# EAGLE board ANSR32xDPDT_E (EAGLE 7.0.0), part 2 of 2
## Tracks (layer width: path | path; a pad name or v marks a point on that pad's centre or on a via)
GND  (via drill 0.5, 0.9)
  Top 0.254: 289.56,74.82 289.56,76.85 288.93,77.48 | FOR_NANO.GND@1 289.56,69.86 | 284.48,93.99 284.48,87.01
  Top 0.406: C1.2 C4.2 | C3.2 C2.2
  Top 1.016: 289.56,67.45 289.56,73.67 289.56,74.82
  Bottom 0.254: 284.48,88.91 FOR_NANO.GND
  other vias: 226.06,82.56 105.41,82.56 274.95,83.2 311.79,83.83 285.12,84.09 315.6,83.83 299.08,80.02 300.48,76.47 281.56,62.62
  pour Top (isolate 0.305): 322.26,43.83 309.56,43.83 309.56,57.16 322.26,57.16
  pour Top (isolate 0.305): -3.17,95.26 321.31,95.26 321.31,57.16 -3.17,57.16
  pour Bottom (isolate 0.305): -5.08,57.16 -5.08,95.26 321.31,95.26 321.31,57.16
  pour Top (isolate 0.305): 323.53,22.87 309.56,22.87 309.56,55.89 323.53,55.89
  pour Top: 320.99,22.87 310.2,22.87 310.2,55.89 320.99,55.89
I2C_SCL  (via drill 0.5, 0.6, 0.9)
  Top 0.254: v274.95,88.28 268.61,88.28 267.97,87.64 v267.97,78.75 | X26.4 294.26,77.48 294.26,78.12 293.24,79.13 291.08,79.13 290.85,79.37 RN26.3 290.83,83.01 290.83,81.29 v290.19,81.29
  Top 0.305: IC2.12 102.87,78.38 103.77,77.48 106.68,77.48 v107.95,78.75 | v223.52,79.39 IC1.12
  Top 0.406: v274.95,88.28 278.13,88.28 278.76,87.64 278.76,84.47 280.67,82.56 v281.94,82.56
  Bottom 0.254: FOR_NANO.A5 297.18,83.83 303.53,77.48 X26.4
  Bottom 0.305: v267.97,78.75 224.16,78.75 v223.52,79.39 221.62,79.39 220.34,78.12 194.94,78.12 194.31,78.75 110.49,78.75 109.86,79.39 108.58,79.39 v107.95,78.75
  Bottom 0.406: v281.94,82.56 288.93,82.56 v290.19,81.29
I2C_SDA  (via drill 0.5, 0.6, 0.9)
  Top 0.254: v274.95,90.82 267.97,90.82 266.7,89.55 v266.7,77.48 | RN26.4 291.65,82.63 v292.35,81.93 | v292.98,77.47 v292.99,77.48 | X26.3 303.53,80.02 302.26,78.75 v295.27,78.75
  Top 0.305: IC2.13 101.6,77.87 103.25,76.21 107.31,76.21 v109.22,78.12 | v222.25,78.12 IC1.13
  Top 0.406: v274.95,90.82 278.76,90.82 280.04,89.55 280.04,87.01 v281.94,85.1
  Bottom 0.254: v292.35,81.93 292.35,78.12 v292.99,77.48 294.26,78.75 v295.27,78.75 | FOR_NANO.A4 299.72,85.74 305.44,80.02 X26.3
  Bottom 0.305: v109.22,78.12 193.68,78.12 194.31,77.48 221.62,77.48 v222.25,78.12 266.06,78.12 v266.7,77.48
  Bottom 0.406: v281.94,85.1 289.58,85.1 RN26.4 291.65,82.63 v292.35,81.93
N$1
  Bottom 1.27: X1.5 306.07,128.92 306.07,122.11 K9.P2
N$2
  Bottom 1.27: X1.6 304.17,125.74 304.17,119.04 K9.O2
N$3
  Top 2.54: X1.4 308.61,124.83 K9.S2
N$4
  Top 1.27: K9.P1 300.69,119.7 297.81,122.57 297.81,125.74 300.99,128.92 300.99,135.27
  Top 2.54: X1.2 300.99,135.27
N$5
  Top 1.27: K9.O1 300.58,114.72 295.91,119.39 295.91,135.27
  Top 2.54: X1.3 295.91,135.27
N$6
  Top 1.27: 306.07,135.27 306.07,130.19 306.07,129.55 306.07,127.65 303.12,124.7 K9.S1
  Top 2.54: X1.1 306.07,135.27
N$7
  Bottom 1.27: X2.5 290.83,128.92 290.83,122.11 K10.P2
N$8
  Bottom 1.27: X2.6 288.93,125.74 288.93,119.04 K10.O2
N$9
  Top 2.54: X2.4 293.37,124.83 K10.S2
N$10
  Top 1.27: 290.83,135.27 290.83,130.19 290.83,129.55 290.83,127.65 287.88,124.7 K10.S1
  Top 2.54: X2.1 290.83,135.27
N$11
  Top 1.27: K10.P1 285.44,119.7 282.57,122.57 282.57,125.74 285.75,128.92 285.75,135.27
  Top 2.54: X2.2 285.75,135.27
N$12
  Top 1.27: K10.O1 285.34,114.72 280.67,119.39 280.67,135.27
  Top 2.54: X2.3 280.67,135.27
N$13
  Bottom 1.27: X3.5 275.59,128.92 275.59,122.11 K11.P2
N$14
  Bottom 1.27: X3.6 273.69,125.74 273.69,119.04 K11.O2
N$15
  Bottom 1.27: X4.5 260.35,128.92 260.35,122.11 K12.P2
N$16
  Bottom 1.27: X4.6 258.44,125.74 258.44,119.04 K12.O2
N$17
  Top 2.54: X3.4 278.13,124.83 K11.S2
N$18
  Top 2.54: X4.4 262.89,124.83 K12.S2
N$19
  Top 1.27: K11.O1 270.1,114.72 265.43,119.39 265.43,135.27
  Top 2.54: X3.3 265.43,135.27
N$20
  Top 1.27: K12.O1 254.86,114.72 250.19,119.39 250.19,135.27
  Top 2.54: X4.3 250.19,135.27
N$21
  Top 1.27: K12.P1 254.97,119.7 252.09,122.57 252.09,125.74 255.27,128.92 255.27,135.27
  Top 2.54: X4.2 255.27,135.27
N$22
  Top 1.27: K11.P1 270.2,119.7 267.33,122.57 267.33,125.74 270.51,128.92 270.51,135.27
  Top 2.54: X3.2 270.51,135.27
N$23
  Top 1.27: 275.59,135.27 275.59,127.65 272.64,124.7 K11.S1
  Top 2.54: X3.1 275.59,135.27
N$24
  Top 1.27: 260.35,135.27 260.35,127.65 257.4,124.7 K12.S1
  Top 2.54: X4.1 260.35,135.27
N$25
  Bottom 1.27: X5.6 226.06,125.74 226.06,119.04 K13.O2
N$26
  Bottom 1.27: X5.5 227.97,128.92 227.97,122.11 K13.P2
N$27
  Top 2.54: X5.4 230.5,124.83 K13.S2
N$28
  Top 1.27: K13.P1 222.58,119.7 219.71,122.57 219.71,125.74 222.88,128.92 222.88,135.27
  Top 2.54: X5.2 222.88,135.27
N$29
  Top 1.27: 227.97,135.27 227.97,127.65 225.02,124.7 K13.S1
  Top 2.54: X5.1 227.97,135.27
N$30
  Top 1.27: K13.O1 222.48,114.72 217.81,119.39 217.81,135.27
  Top 2.54: X5.3 217.81,135.27
N$31
  Bottom 1.27: X6.5 212.72,128.92 212.72,122.11 K14.P2
N$32
  Bottom 1.27: X6.6 210.82,125.74 210.82,119.04 K14.O2
N$33
  Top 1.27: K14.P1 207.34,119.7 204.47,122.57 204.47,125.74 207.65,128.92 207.65,135.27
  Top 2.54: X6.2 207.65,135.27
N$34
  Top 1.27: 212.72,135.27 212.72,127.65 209.78,124.7 K14.S1
  Top 2.54: X6.1 212.72,135.27
N$35
  Top 1.27: K15.P1 192.1,119.7 189.23,122.57 189.23,125.74 192.41,128.92 192.41,135.27
  Top 2.54: X7.2 192.41,135.27
N$36
  Top 1.27: K16.P1 176.86,119.7 173.99,122.57 173.99,125.74 177.16,128.92 177.16,135.27
  Top 2.54: X8.2 177.16,135.27
N$37
  Bottom 1.27: X8.5 182.25,128.92 182.25,122.11 K16.P2
N$38
  Bottom 1.27: X8.6 180.34,125.74 180.34,119.04 K16.O2
N$39
  Top 1.27: K14.O1 207.65,114.95 202.56,120.03 202.56,135.27
  Top 2.54: X6.3 202.56,135.27
N$40
  Top 1.27: K16.O1 176.76,114.72 172.09,119.39 172.09,135.27
  Top 2.54: X8.3 172.09,135.27
N$41
  Top 1.27: K15.O1 192,114.72 187.32,119.39 187.32,135.27
  Top 2.54: X7.3 187.32,135.27
N$42
  Bottom 1.27: X7.6 195.58,125.74 195.58,119.04 K15.O2
N$43
  Bottom 1.27: X7.5 197.49,128.92 197.49,122.11 K15.P2
N$44
  Top 2.54: X6.4 215.26,124.83 K14.S2
N$45
  Top 2.54: X7.4 200.03,124.83 K15.S2
N$46
  Top 1.27: 197.49,135.27 197.49,127.65 194.54,124.7 K15.S1
  Top 2.54: X7.1 197.49,135.27
N$47
  Top 1.27: 182.25,135.27 182.25,127.65 179.3,124.7 K16.S1
  Top 2.54: X8.1 182.25,135.27
N$48
  Top 2.54: X8.4 184.78,124.83 K16.S2
N$49
  Bottom 1.27: X9.5 139.7,23.51 139.7,30.31 K17.P2
N$50
  Bottom 1.27: X9.6 141.6,26.05 141.6,33.39 K17.O2
N$51
  Top 2.54: X9.4 137.16,27.6 K17.S2
N$52
  Top 1.27: 144.78,17.16 144.78,23.51 147.96,26.68 147.96,29.55 K17.P1
  Top 2.54: X9.2 144.78,17.16
N$53
  Top 1.27: 149.86,17.16 149.86,32.63 K17.O1
  Top 2.54: X9.3 149.86,17.16
N$54
  Top 1.27: K17.S1 144.78,27.32 142.88,27.32 139.7,24.14 139.7,17.16
  Top 2.54: X9.1 139.7,17.16
N$55
  Bottom 1.27: X10.5 127,21.6 124.46,24.14 124.46,30.31 K18.P2
N$56
  Bottom 1.27: X10.6 126.36,26.68 126.36,33.39 K18.O2
N$57
  Top 2.54: X10.4 121.92,27.6 K18.S2
N$58
  Top 1.27: 124.46,17.16 124.46,24.78 127.41,27.72 K18.S1
  Top 2.54: X10.1 124.46,17.16
N$59
  Top 1.27: 129.54,17.16 129.54,23.51 132.72,26.68 132.72,29.55 K18.P1
  Top 2.54: X10.2 129.54,17.16
N$60
  Top 1.27: 134.62,17.16 134.62,32.63 K18.O1
  Top 2.54: X10.3 134.62,17.16
N$61
  Bottom 1.27: X11.5 109.22,23.51 109.22,30.31 K19.P2
N$62
  Bottom 1.27: X11.6 111.12,26.68 111.12,33.39 K19.O2
N$63
  Bottom 1.27: X12.5 93.98,23.51 93.98,30.31 K20.P2
N$64
  Bottom 1.27: X12.6 95.89,26.68 95.89,33.39 K20.O2
N$65
  Top 2.54: X11.4 106.68,27.6 K19.S2
N$66
  Top 2.54: X12.4 91.44,27.6 K20.S2
N$67
  Top 1.27: 119.38,17.16 119.38,32.63 K19.O1
  Top 2.54: X11.3 119.38,17.16
N$68
  Top 1.27: 104.14,17.16 104.14,32.63 K20.O1
  Top 2.54: X12.3 104.14,17.16
N$69
  Top 1.27: 99.06,17.16 99.06,23.51 102.23,26.68 102.23,29.55 K20.P1
  Top 2.54: X12.2 99.06,17.16
N$70
  Top 1.27: 114.3,17.16 114.3,23.51 117.47,26.68 117.47,29.55 K19.P1
  Top 2.54: X11.2 114.3,17.16
N$71
  Top 1.27: 109.22,17.16 109.22,24.78 112.17,27.72 K19.S1
  Top 2.54: X11.1 109.22,17.16
N$72
  Top 1.27: K20.S1 99.06,27.32 97.16,27.32 93.98,24.14 93.98,17.16
  Top 2.54: X12.1 93.98,17.16
N$73
  Bottom 1.27: X13.6 63.5,26.68 63.5,33.39 K21.O2
N$74
  Bottom 1.27: X13.5 61.59,23.51 61.59,30.31 K21.P2
N$75
  Top 2.54: X13.4 59.05,27.6 K21.S2
N$76
  Top 1.27: K21.P1 66.98,32.73 69.85,29.86 69.85,26.68 66.67,23.51 66.67,17.16
  Top 2.54: X13.2 66.67,17.16
N$77
  Top 1.27: K21.S1 66.67,27.32 64.77,27.32 61.59,24.14 61.59,17.16
  Top 2.54: X13.1 61.59,17.16
N$78
  Top 1.27: 71.75,17.16 71.75,32.63 K21.O1
  Top 2.54: X13.3 71.75,17.16
N$79
  Bottom 1.27: X14.5 46.35,23.51 46.35,30.31 K22.P2
N$80
  Bottom 1.27: X14.6 48.26,26.68 48.26,33.39 K22.O2
N$81
  Top 1.27: K22.P1 51.74,32.73 54.61,29.86 54.61,26.68 51.44,23.51 51.44,17.16
  Top 2.54: X14.2 51.44,17.16
N$82
  Top 1.27: K22.S1 51.44,27.32 49.53,27.32 46.35,24.14 46.35,17.16
  Top 2.54: X14.1 46.35,17.16
N$83
  Top 1.27: 36.2,17.16 36.2,23.51 39.37,26.68 39.37,29.55 K23.P1
  Top 2.54: X15.2 36.2,17.16
N$84
  Top 1.27: 20.95,17.16 20.95,23.51 24.13,26.68 24.13,29.55 K24.P1
  Top 2.54: X16.2 20.95,17.16
N$85
  Bottom 1.27: X16.5 15.88,23.51 15.88,30.31 K24.P2
N$86
  Bottom 1.27: X16.6 17.78,26.68 17.78,33.39 K24.O2
N$87
  Top 1.27: K22.O1 51.84,37.71 56.52,33.03 56.52,17.16
  Top 2.54: X14.3 56.52,17.16
N$88
  Top 1.27: 26.04,17.16 26.04,32.63 K24.O1
  Top 2.54: X16.3 26.04,17.16
N$89
  Top 1.27: 41.27,17.16 41.27,32.63 K23.O1
  Top 2.54: X15.3 41.27,17.16
N$90
  Bottom 1.27: X15.6 33.02,26.68 33.02,33.39 K23.O2
N$91
  Bottom 1.27: X15.5 31.11,23.51 31.11,30.31 K23.P2
N$92
  Top 2.54: X14.4 43.81,27.6 K22.S2
N$93
  Top 2.54: X15.4 28.57,27.6 K23.S2
N$94
  Top 1.27: 31.11,17.16 31.11,20.97 31.11,22.64 31.11,24.14 34.7,27.72 K23.S1
  Top 2.54: X15.1 31.11,17.16
N$95
  Top 1.27: 15.88,17.16 15.88,24.14 19.05,27.32 20.32,27.32 20.73,27.72 K24.S1
  Top 2.54: X16.1 15.88,17.16
N$96
  Top 2.54: X16.4 13.34,27.6 K24.S2
N$97
  Bottom 1.27: X17.5 149.86,128.92 149.86,122.11 K25.P2
N$98
  Bottom 1.27: X17.6 147.96,125.74 147.96,119.04 K25.O2
N$99
  Top 2.54: X17.4 152.4,124.83 K25.S2
N$100
  Top 1.27: K25.P1 144.47,119.7 141.6,122.57 141.6,125.74 144.78,128.92 144.78,135.27
  Top 2.54: X17.2 144.78,135.27
N$101
  Top 1.27: K25.O1 144.78,114.95 139.7,120.03 139.7,135.27
  Top 2.54: X17.3 139.7,135.27
N$102
  Top 1.27: 149.86,135.27 149.86,128.28 146.28,124.7 K25.S1
  Top 2.54: X17.1 149.86,135.27
N$103
  Bottom 1.27: X18.5 134.62,128.92 134.62,122.11 K26.P2
N$104
  Bottom 1.27: X18.6 132.72,125.74 132.72,119.04 K26.O2
N$105
  Top 2.54: X18.4 137.16,124.83 K26.S2
N$106
  Top 1.27: 134.62,135.27 134.62,128.28 131.04,124.7 K26.S1
  Top 2.54: X18.1 134.62,135.27
N$107
  Top 1.27: K26.P1 129.24,119.7 126.36,122.57 126.36,125.74 129.54,128.92 129.54,135.27
  Top 2.54: X18.2 129.54,135.27
N$108
  Top 1.27: K26.O1 129.54,114.95 124.46,120.03 124.46,135.27
  Top 2.54: X18.3 124.46,135.27
N$109
  Bottom 1.27: X19.5 119.38,128.92 119.38,122.11 K27.P2
N$110
  Bottom 1.27: X19.6 117.47,125.74 117.47,119.04 K27.O2
N$111
  Bottom 1.27: X20.5 104.14,128.92 104.14,122.11 K28.P2
N$112
  Bottom 1.27: X20.6 102.23,125.74 102.23,119.04 K28.O2
N$113
  Top 2.54: X19.4 121.92,124.83 K27.S2
N$114
  Top 2.54: X20.4 106.68,124.83 K28.S2
N$115
  Top 1.27: K27.O1 113.89,114.72 109.22,119.39 109.22,135.27
  Top 2.54: X19.3 109.22,135.27
N$116
  Top 1.27: K28.O1 98.65,114.72 93.98,119.39 93.98,135.27
  Top 2.54: X20.3 93.98,135.27
N$117
  Top 1.27: K28.P1 98.75,119.7 95.89,122.57 95.89,125.74 99.06,128.92 99.06,135.27
  Top 2.54: X20.2 99.06,135.27
N$118
  Top 1.27: K27.P1 113.36,119.7 111.12,121.93 111.12,125.74 114.3,128.92 114.3,135.27
  Top 2.54: X19.2 114.3,135.27
N$119
  Top 1.27: 119.38,135.27 119.38,128.28 115.8,124.7 K27.S1
  Top 2.54: X19.1 119.38,135.27
N$120
  Top 1.27: 104.14,135.27 104.14,128.28 100.56,124.7 K28.S1
  Top 2.54: X20.1 104.14,135.27
N$121
  Bottom 1.27: K29.O2 73.89,114.72 69.85,118.76 69.85,125.74 X21.6
N$122
  Bottom 1.27: K29.P2 73.99,119.7 71.75,121.93 71.75,128.92 X21.5
N$123
  Top 2.54: X21.4 74.3,124.83 K29.S2
N$124
  Top 1.27: K29.P1 66.37,119.7 63.5,122.57 63.5,125.74 66.67,128.92 66.67,135.27
  Top 2.54: X21.2 66.67,135.27
N$125
  Top 1.27: 71.75,135.27 71.75,128.28 68.17,124.7 K29.S1
  Top 2.54: X21.1 71.75,135.27
N$126
  Top 1.27: K29.O1 66.27,114.72 61.59,119.39 61.59,135.27
  Top 2.54: X21.3 61.59,135.27
N$127
  Bottom 1.27: K30.P2 58.93,120.15 56.52,122.57 56.52,128.92 X22.5
N$128
  Bottom 1.27: K30.O2 58.65,114.72 54.61,118.76 54.61,125.74 X22.6
N$129
  Top 1.27: K30.P1 51.13,119.7 48.26,122.57 48.26,125.74 51.44,128.92 51.44,135.27
  Top 2.54: X22.2 51.44,135.27
N$130
  Top 1.27: 56.52,135.27 56.52,128.28 52.93,124.7 K30.S1
  Top 2.54: X22.1 56.52,135.27
N$131
  Top 1.27: K31.P1 36.2,120.03 33.02,123.2 33.02,125.74 36.2,128.92 36.2,135.27
  Top 2.54: X23.2 36.2,135.27
N$132
  Top 1.27: K32.P1 20.95,120.03 17.78,123.2 17.78,125.74 20.95,128.92 20.95,135.27
  Top 2.54: X24.2 20.95,135.27
N$133
  Bottom 1.27: K32.P2 28.45,120.15 26.04,122.57 26.04,128.92 X24.5
N$134
  Bottom 1.27: K32.O2 28.17,114.72 24.13,118.76 24.13,125.74 X24.6
N$135
  Top 1.27: K30.O1 51.03,114.72 46.35,119.39 46.35,135.27
  Top 2.54: X22.3 46.35,135.27
N$136
  Top 1.27: K32.O1 20.55,114.72 15.88,119.39 15.88,135.27
  Top 2.54: X24.3 15.88,135.27
N$137
  Top 1.27: K31.O1 36.2,114.95 31.11,120.03 31.11,135.27
  Top 2.54: X23.3 31.11,135.27
N$138
  Bottom 1.27: K31.O2 43.69,115.07 39.37,119.39 39.37,125.74 X23.6
N$139
  Bottom 1.27: K31.P2 43.69,120.15 41.27,122.57 41.27,128.92 X23.5
N$140
  Top 2.54: X22.4 59.05,124.83 K30.S2
N$141
  Top 2.54: X23.4 43.81,124.83 K31.S2
N$142
  Top 1.27: 41.27,135.27 41.27,128.28 37.69,124.7 K31.S1
  Top 2.54: X23.1 41.27,135.27
N$143
  Top 1.27: 26.04,135.27 26.04,128.28 22.45,124.7 K32.S1
  Top 2.54: X24.1 26.04,135.27
N$144
  Top 2.54: X24.4 28.57,124.83 K32.S2
N$163
  Top 0.254: POWER1.A 317.11,30.61 316.74,30.24 315.46,30.24 RNB1.3
  Top 0.406: 315.42,30.37 RNB1.3
N$164
  Top 0.813: 282.57,66.18 IC7.8 291.01,66.18 H1.2 | 282.57,66.18 280.8,66.18 280.04,65.42 280.04,60.87 279.53,60.36 279.53,58.96 D1.C 279.38,58.81 277.37,58.81 276.48,59.7 269.24,59.7 268.35,60.59 CD1.2 | 282.55,66.2 282.57,66.18
N$165
  Top 0.813: CD1.1 270.66,67.17 271.78,66.05 276.61,66.05 276.73,66.18 IC7.1
N$203
  Bottom 1.27: X28.5 295.91,23.51 295.91,30.31 K1.P2
N$204
  Bottom 1.27: X28.6 297.81,26.05 297.81,32.75 K1.O2
N$205
  Top 2.54: X28.4 293.37,27.6 K1.S2
N$206
  Top 1.27: K1.P1 301.3,32.73 304.17,29.86 304.17,26.68 300.99,23.51 300.99,17.16
  Top 2.54: X28.2 300.99,17.16
N$207
  Top 1.27: K1.O1 300.99,37.48 306.07,32.4 306.07,17.16
  Top 2.54: X28.3 306.07,17.16
N$208
  Top 1.27: 295.91,17.16 295.91,24.78 298.86,27.72 K1.S1
  Top 2.54: X28.1 295.91,17.16
N$209
  Bottom 1.27: X29.5 280.67,23.51 280.67,30.31 K2.P2
N$210
  Bottom 1.27: X29.6 282.57,26.68 282.57,33.39 K2.O2
N$211
  Top 2.54: X29.4 278.13,27.6 K2.S2
N$212
  Top 1.27: K2.S1 285.75,27.32 283.85,27.32 280.67,24.14 280.67,17.16
  Top 2.54: X29.1 280.67,17.16
N$213
  Top 1.27: K2.P1 286.06,32.73 288.93,29.86 288.93,26.68 285.75,23.51 285.75,17.16
  Top 2.54: X29.2 285.75,17.16
N$214
  Top 1.27: K2.O1 285.75,37.48 290.83,32.4 290.83,17.16
  Top 2.54: X29.3 290.83,17.16
N$215
  Bottom 1.27: X30.5 265.43,23.51 265.43,30.31 K3.P2
N$216
  Bottom 1.27: X30.6 267.33,26.68 267.33,33.39 K3.O2
N$217
  Bottom 1.27: X31.5 252.09,20.97 250.19,22.87 250.19,30.31 K4.P2
N$218
  Bottom 1.27: X31.6 252.09,26.68 252.09,33.39 K4.O2
N$219
  Top 2.54: X30.4 262.89,27.6 K3.S2
N$220
  Top 2.54: X31.4 247.78,20.97 K4.S2
N$221
  Top 1.27: K3.O1 270.92,37.71 275.59,33.03 275.59,17.16
  Top 2.54: X30.3 275.59,17.16
N$222
  Top 1.27: 260.35,17.16 260.35,32.63 K4.O1
  Top 2.54: X31.3 260.35,17.16
N$223
  Top 1.27: K4.P1 255.27,32.4 258.44,29.22 258.44,26.68 255.27,23.51 255.27,17.16
  Top 2.54: 255.27,17.16 X31.2
N$224
  Top 1.27: 270.51,17.16 270.51,23.51 273.69,26.68 273.74,29.48 273.38,29.86 K3.P1
  Top 2.54: X30.2 270.51,17.16
N$225
  Top 1.27: 265.43,17.16 265.43,24.78 268.38,27.72 K3.S1
  Top 2.54: X30.1 265.43,17.16
N$226
  Top 1.27: 250.19,17.16 250.19,24.78 253.14,27.72 K4.S1
  Top 2.54: X31.1 250.19,17.16
N$304
  Bottom 1.27: X32.6 219.71,26.68 219.71,33.39 K5.O2
N$305
  Bottom 1.27: X32.5 217.81,23.51 217.81,30.31 K5.P2
N$306
  Top 2.54: X32.4 215.26,27.6 K5.S2
N$307
  Top 1.27: 222.88,17.16 222.88,23.51 226.06,26.68 226.06,29.55 K5.P1
  Top 2.54: X32.2 222.88,17.16
N$308
  Top 1.27: 217.81,17.16 217.81,24.78 220.75,27.72 K5.S1
  Top 2.54: X32.1 217.81,17.16
N$309
  Top 1.27: 227.97,17.16 227.97,32.63 K5.O1
  Top 2.54: X32.3 227.97,17.16
N$310
  Bottom 1.27: X33.5 202.56,23.51 202.56,30.31 K6.P2
N$311
  Bottom 1.27: X33.6 204.47,26.68 204.47,33.39 K6.O2
N$312
  Top 1.27: 207.65,17.16 207.65,23.51 210.82,26.68 210.82,29.55 K6.P1
  Top 2.54: X33.2 207.65,17.16
N$313
  Top 1.27: 202.56,17.16 202.56,24.78 205.51,27.72 K6.S1
  Top 2.54: X33.1 202.56,17.16
N$314
  Top 1.27: 192.41,17.16 192.41,23.51 195.58,26.68 195.58,29.55 K7.P1
  Top 2.54: X34.2 192.41,17.16
N$315
  Top 1.27: 177.16,17.16 177.16,23.51 180.34,26.68 180.34,29.55 K8.P1
  Top 2.54: X35.2 177.16,17.16
N$316
  Bottom 1.27: X35.5 172.09,23.51 172.09,30.31 K8.P2
N$317
  Bottom 1.27: X35.6 173.99,26.68 173.99,33.39 K8.O2
N$318
  Top 1.27: 212.72,17.16 212.72,32.63 K6.O1
  Top 2.54: X33.3 212.72,17.16
N$319
  Top 1.27: 182.25,17.16 182.25,32.63 K8.O1
  Top 2.54: X35.3 182.25,17.16
N$320
  Top 1.27: 197.49,17.16 197.49,32.63 K7.O1
  Top 2.54: X34.3 197.49,17.16
N$321
  Bottom 1.27: X34.6 189.23,26.68 189.23,33.39 K7.O2
N$322
  Bottom 1.27: X34.5 187.32,23.51 187.32,30.31 K7.P2
N$323
  Top 2.54: X33.4 200.03,27.6 K6.S2
N$324
  Top 2.54: X34.4 184.78,27.6 K7.S2
N$325
  Top 1.27: 187.32,17.16 187.32,24.78 190.27,27.72 K7.S1
  Top 2.54: X34.1 187.32,17.16
N$326
  Top 1.27: 172.09,17.16 172.09,24.78 175.03,27.72 K8.S1
  Top 2.54: X35.1 172.09,17.16
N$327
  Top 2.54: X35.4 169.54,27.6 K8.S2
N$405  (via drill 0.5)
  Top 0.229: IC1.21 228.6,70.81 227.97,70.18 214.63,70.18 214,70.81 IC3.1
  Top 0.254: 228.6,70.81 v228.6,73.29 | v242.82,70.37 243.46,69.74 245.52,69.74
  Top 0.305: 245.52,69.74 245.58,69.74 RN19.5
  Bottom 0.229: v228.6,73.29 228.6,73.04 229.24,73.67 242.19,73.67 242.82,73.04 v242.82,70.37
N$406  (via drill 0.5)
  Top 0.229: IC1.25 v233.68,69.99 233.68,68.28 233.04,67.64 209.55,67.64 208.91,68.28 IC3.5 | v239.4,66.37 242.89,66.37 243.21,66.05 245.51,66.05 RN18.5
  Bottom 0.229: v233.68,69.99 233.68,71.28 234.04,71.64 238.99,71.64 239.4,71.24 v239.4,66.37
N$407  (via drill 0.5)
  Top 0.229: IC1.26 v234.95,69.99 234.95,67.96 234,67.01 208.28,67.01 207.65,67.64 IC3.6 | v240.35,65.42 242.89,65.42 243.21,65.1 245.5,65.1 RN18.6
  Bottom 0.229: v234.95,69.99 234.95,71.01 235.08,71.13 238.25,71.13 238.38,71.01 238.38,65.67 238.63,65.42 v240.35,65.42
N$408  (via drill 0.6)
  Top 0.305: IC2.16 v101.6,74.94 | v222.25,73.67 IC1.16 | RN17.6 264.05,82.16 | U$13.A1 264.8,90.18 265.43,89.55 265.43,82.56 265.03,82.16 264.05,82.16 | 264.05,82.16 264.92,81.29 v264.92,74.31
  Bottom 0.305: v101.6,74.94 102.87,76.21 110.49,76.21 111.12,76.85 192.41,76.85 193.04,76.21 219.07,76.21 221.62,73.67 v222.25,73.67 222.88,74.31 v264.92,74.31
N$409  (via drill 0.5)
  Top 0.229: IC1.22 229.87,70.18 229.24,69.54 213.36,69.54 212.72,70.18 IC3.2
  Top 0.254: 229.87,70.18 v229.87,69.99 | v241.81,69.61 242.32,69.61 242.95,68.97 245.56,68.97 RN19.6
  Bottom 0.229: v229.87,69.99 229.87,72.78 230.25,73.16 241.3,73.16 241.81,72.66 v241.81,69.61
N$410  (via drill 0.5)
  Top 0.229: IC1.23 231.14,69.54 230.5,68.91 212.09,68.91 211.46,69.54 IC3.3
  Top 0.254: 231.14,69.54 v231.14,69.99 | v240.92,68.59 241.55,68.59 241.94,68.21 245.56,68.21 RN19.7
  Bottom 0.229: v231.14,69.99 231.14,72.4 231.39,72.66 240.54,72.66 240.92,72.28 v240.92,68.59
  Bottom 0.254: 241.17,68.47 v240.92,68.59
N$411  (via drill 0.5)
  Top 0.229: IC1.24 232.41,68.91 231.78,68.28 210.82,68.28 210.19,68.91 IC3.4
  Top 0.254: 232.41,68.91 v232.41,69.99 | v240.54,67.32 245.51,67.32 RN19.8
  Bottom 0.229: v232.41,69.99 232.41,71.64 232.92,72.15 239.27,72.15 240.03,71.39 240.03,67.83 v240.54,67.32
N$416  (via drill 0.6)
  Top 0.203: 212.72,79.39 213.04,79.7 218.76,79.7 219.71,80.66 219.71,82.88 220.34,83.51 236.85,83.51 237.49,84.15 v237.49,88.91
  Top 0.229: v237.49,88.91 237.49,89.8 236.73,90.56 236.73,91.34 RN21.8
  Top 0.406: v237.49,82.56 IC1.1 | IC4.8 212.72,79.39
  Bottom 0.406: v237.49,88.91 v237.49,82.56
N$417  (via drill 0.6)
  Top 0.203: IC4.7 211.46,79.7 211.96,80.21 218.25,80.21 219.07,81.04 219.07,83.51 219.71,84.15 235.59,84.15 236.22,84.78 v236.22,88.91
  Top 0.229: v236.22,88.91 236.22,89.93 235.84,90.31 235.84,91.4 RN21.7
  Top 0.406: v236.22,82.56 IC1.2
  Bottom 0.406: v236.22,88.91 v236.22,82.56
N$418  (via drill 0.6)
  Top 0.203: IC4.6 210.19,80.02 210.88,80.72 217.49,80.72 218.44,81.67 218.44,84.15 219.07,84.78 234.31,84.78 234.95,85.42 v234.95,88.91
  Top 0.229: v234.95,88.91 234.95,90.44 235.08,90.56 235.08,91.4 RN21.6
  Top 0.406: v234.95,82.56 IC1.3
  Bottom 0.406: v234.95,88.91 v234.95,82.56
N$419  (via drill 0.6)
  Top 0.203: IC4.5 208.91,80.02 210.12,81.23 216.85,81.23 217.81,82.18 217.81,84.78 218.44,85.42 233.04,85.42 233.68,86.06 v233.68,88.91
  Top 0.229: v233.68,88.91 233.68,90.06 234.19,90.56 234.19,91.34 RN21.5
  Top 0.406: v233.68,82.56 IC1.4
  Bottom 0.406: v233.68,82.56 v233.68,88.91
N$420  (via drill 0.6)
  Top 0.203: IC4.4 207.65,80.02 209.36,81.74 216.34,81.74 217.17,82.56 217.17,85.42 217.81,86.06 231.78,86.06 232.41,86.69 v232.41,88.91
  Top 0.229: v232.41,88.91 232.41,89.67 231.78,90.31 231.78,91.34 RN20.8
  Top 0.406: v232.41,82.56 IC1.5
  Bottom 0.406: v232.41,88.91 v232.41,82.56
N$421  (via drill 0.6)
  Top 0.203: IC4.3 206.38,80.02 208.6,82.25 215.84,82.25 216.53,82.94 216.53,86.06 217.17,86.69 230.5,86.69 231.14,87.32 v231.14,88.91
  Top 0.229: v231.14,88.91 231.14,90.06 230.89,90.31 230.89,91.4 RN20.7
  Top 0.406: v231.14,82.56 IC1.6
  Bottom 0.406: v231.14,88.91 v231.14,82.56
N$422  (via drill 0.6)
  Top 0.203: IC4.2 205.1,80.02 207.84,82.75 215.2,82.75 215.9,83.45 215.9,86.69 216.53,87.32 229.42,87.32 229.87,87.77 v229.87,88.91
  Top 0.229: IC1.7 229.87,80.66 | v229.87,88.91 229.87,89.93 230.12,90.18 230.12,91.4 RN20.6
  Top 0.406: 229.87,88.54 v229.87,88.91 | v229.87,82.56 IC1.7
  Bottom 0.406: v229.87,88.91 v229.87,82.56
N$423  (via drill 0.6)
  Top 0.203: IC4.1 203.84,80.02 207.2,83.39 214.69,83.39 215.26,83.96 215.26,87.25 215.97,87.96 228.15,87.96 228.6,88.41 v228.6,88.91
  Top 0.229: v228.6,88.91 228.6,89.93 229.24,90.56 229.24,91.34 RN20.5
  Top 0.406: v228.6,82.56 IC1.8
  Bottom 0.406: v228.6,82.56 v228.6,88.91
N$424  (via drill 0.5)
  Top 0.229: IC2.21 v107.95,73.23 107.95,70.76 107.56,70.37 94.61,70.37 93.98,71.01 IC5.1 | v123.19,67.32 124.86,67.32 RN22.5
  Bottom 0.229: v107.95,73.23 107.95,74.31 108.58,74.94 122.56,74.94 123.19,74.31 v123.19,67.32
N$425  (via drill 0.5)
  Top 0.229: IC5.2 92.71,70.5 93.34,69.86 109.22,69.86 v109.22,70.05 IC2.22 | RN22.6 122,66.45 v121.92,66.37
  Bottom 0.229: v121.92,66.37 121.92,73.67 121.28,74.31 109.86,74.31 109.22,73.67 v109.22,70.05
N$426  (via drill 0.5)
  Top 0.229: IC5.3 91.44,69.86 92.08,69.23 109.98,69.23 110.49,69.74 v110.49,70.05 IC2.23 | RN22.7 122.79,65.65 122.56,65.42 v120.65,65.42
  Bottom 0.229: v120.65,65.42 120.65,73.04 120.02,73.67 111.12,73.67 110.49,73.04 v110.49,70.05
N$427  (via drill 0.5)
  Top 0.229: IC5.4 90.17,69.23 90.81,68.59 111.12,68.59 111.76,69.23 v111.76,70.05 IC2.24 | RN22.8 122.94,64.85 122.56,64.47 119.7,64.47 v119.06,65.1
  Bottom 0.229: v119.06,65.1 119.06,72.33 118.35,73.04 112.39,73.04 111.76,72.4 v111.76,70.05
N$428  (via drill 0.5)
  Top 0.229: IC5.5 88.9,68.59 89.53,67.96 112.39,67.96 113.03,68.59 v113.03,70.05 IC2.25 | RN23.5 122.94,63.44 v122.87,63.51
  Bottom 0.229: v122.87,63.51 119.06,63.51 118.11,64.47 118.11,71.77 117.47,72.4 113.67,72.4 113.03,71.77 v113.03,70.05
N$429  (via drill 0.5)
  Top 0.229: IC5.6 87.63,67.96 88.27,67.32 113.67,67.32 114.3,67.96 v114.3,70.05 IC2.26 | RN23.6 122,62.64 v121.92,62.56
  Bottom 0.229: v121.92,62.56 118.75,62.56 117.16,64.15 117.16,71.06 116.45,71.77 114.64,71.77 IC2.26 v114.3,70.05
N$430  (via drill 0.5)
  Top 0.229: IC5.7 86.36,67.32 87,66.69 114.94,66.69 115.57,67.32 v115.57,70.05 IC2.27 | RN23.7 122.79,61.84 122.56,61.61 v120.65,61.61
  Bottom 0.229: v120.65,61.61 117.47,61.61 115.57,63.51 v115.57,70.05
N$431
  Top 0.229: IC2.28 116.84,66.69 | 116.84,66.69 116.2,66.05 85.72,66.05 85.09,66.69 IC5.8 | RN23.8 121.67,61.04 121.28,60.65 119.7,60.65 119.38,60.97 119.38,63.51 116.84,66.05 116.84,66.69
N$432  (via drill 0.6)
  Top 0.203: IC6.8 92.71,79.39 93.34,80.02 98.42,80.02 99.06,80.66 99.06,82.56 100.33,83.83 116.2,83.83 116.84,84.47 v116.84,88.91 | v116.84,82.56 IC2.1
  Top 0.229: v116.84,88.91 116.84,89.87 116.2,90.5 116.2,91.22 RN25.8
  Bottom 0.203: v116.84,88.91 v116.84,82.56
N$433  (via drill 0.6)
  Top 0.203: IC6.7 91.44,79.39 92.46,80.4 97.54,80.4 98.42,81.29 98.42,83.2 99.69,84.47 114.94,84.47 115.57,85.1 v115.57,88.91 | v115.57,82.56 IC2.2
  Top 0.229: v115.57,88.91 115.57,90.18 115.25,90.5 115.25,91.2 RN25.7
  Bottom 0.203: v115.57,88.91 v115.57,82.56
N$434  (via drill 0.6)
  Top 0.203: IC6.6 90.17,79.39 91.57,80.78 96.65,80.78 97.79,81.93 97.79,83.83 99.06,85.1 113.67,85.1 114.3,85.74 v114.3,88.91 | v114.3,82.56 IC2.3
  Top 0.229: v114.3,88.91 114.3,90.18 114.62,90.5 114.62,91.2 RN25.6
  Bottom 0.203: v114.3,88.91 v114.3,82.56
N$435  (via drill 0.6)
  Top 0.203: IC6.5 88.9,80.02 90.04,81.17 95.76,81.17 97.16,82.56 97.16,84.47 98.42,85.74 112.39,85.74 113.03,86.37 v113.03,88.91 | v113.03,82.56 IC2.4
  Top 0.229: v113.03,88.91 113.03,89.87 113.67,90.5 113.67,91.22 RN25.5
  Bottom 0.203: v113.03,88.91 v113.03,82.56
N$436  (via drill 0.6)
  Top 0.203: IC6.4 87.63,80.02 89.15,81.55 94.87,81.55 96.52,83.2 96.52,85.1 97.79,86.37 111.12,86.37 111.76,87.01 v111.76,88.91 | v111.76,82.56 IC2.5
  Top 0.229: v111.76,88.91 111.76,89.87 111.12,90.5 111.12,91.22 RN24.8
  Bottom 0.203: v111.76,88.91 v111.76,82.56
N$437  (via drill 0.6)
  Top 0.203: IC6.3 86.36,80.02 88.27,81.93 93.98,81.93 95.89,83.83 95.89,85.74 97.16,87.01 109.86,87.01 110.49,87.64 v110.49,88.91 | v110.49,82.56 IC2.6
  Top 0.229: v110.49,88.91 110.49,90.18 110.17,90.5 110.17,91.2 RN24.7
  Bottom 0.203: v110.49,88.91 v110.49,82.56
N$438  (via drill 0.6)
  Top 0.203: IC6.2 85.09,80.02 87.38,82.31 93.09,82.31 95.25,84.47 95.25,86.37 96.52,87.64 108.58,87.64 109.22,88.28 v109.22,88.91 | v109.22,82.56 IC2.7
  Top 0.229: v109.22,88.91 109.22,90.18 109.54,90.5 109.54,91.2 RN24.6
  Bottom 0.203: v109.22,88.91 v109.22,82.56
N$439  (via drill 0.6)
  Top 0.203: IC6.1 83.82,80.02 86.49,82.69 92.46,82.69 94.61,84.85 94.61,87.01 95.89,88.28 107.31,88.28 v107.95,88.91 | v107.95,82.56 IC2.8
  Top 0.229: v107.95,88.91 107.95,89.87 108.58,90.5 108.58,91.22 RN24.5
  Bottom 0.203: v107.95,88.91 v107.95,82.56
N$440
  Top 0.406: RN2.7 53.74,82.16 52.7,83.2 34.17,83.2 R30.C
N$441
  Top 0.406: RN5.1 184.22,83.76 183.51,84.47 157.37,84.47 R16.C
N$442
  Top 0.406: RN8.7 RN7.2
N$443
  Top 0.406: RN7.3 RN8.6
N$444
  Top 0.406: RN8.5 RN7.4
N$445
  Top 0.406: RN5.2 183.75,82.96 182.88,83.83 160.54,83.83 R15.C
N$446
  Top 0.406: RN4.3 52.47,78.35 50.16,80.66 46.88,80.66 R26.C
N$447
  Top 0.406: RN5.4 182.81,81.36 181.61,82.56 166.89,82.56 R13.C
N$448
  Top 0.406: RN5.5 RN6.4
N$449
  Top 0.406: RN7.1 RN8.8
N$450
  Top 0.406: RN8.1 182.95,79.95 180.97,81.93 170.06,81.93 R12.C
N$451
  Top 0.406: RN5.6 RN6.3
N$452
  Top 0.406: RN8.2 182.48,79.15 180.34,81.29 173.24,81.29 R11.C
N$453
  Top 0.406: RN6.2 RN5.7
N$454
  Top 0.406: RN5.8 RN6.1
N$455
  Top 0.406: RN3.4 RN4.5
N$456
  Top 0.406: RN2.5 54.68,83.76 53.98,84.47 27.82,84.47 R32.C
N$458
  Top 0.406: RN5.3 183.28,82.16 182.25,83.2 163.72,83.2 R14.C
N$459
  Top 0.406: RN8.3 182.01,78.35 179.71,80.66 176.41,80.66 R10.C
N$460
  Top 0.406: RN2.8 53.27,81.36 52.07,82.56 37.35,82.56 R29.C
N$461
  Top 0.406: RN4.1 53.41,79.95 51.44,81.93 40.52,81.93 R28.C
N$462
  Top 0.406: RN4.2 52.94,79.15 50.8,81.29 43.7,81.29 R27.C
N$463
  Top 0.406: RN12.4 RN11.5
N$464
  Top 0.305: R25.C 49.65,79.39
  Top 0.406: RN4.4 52,77.55 50.16,79.39 49.65,79.39
N$465
  Top 0.406: RN2.1 RN1.8
N$466
  Top 0.406: RN2.2 RN1.7
N$467
  Top 0.406: RN2.3 RN1.6
N$468
  Top 0.406: RN2.4 RN1.5
N$469
  Top 0.406: RN2.6 54.21,82.96 53.34,83.83 31,83.83 R31.C
N$470
  Top 0.406: RN8.4 181.54,77.55 179.71,79.39 179.19,79.39 R9.C
N$473
  Top 0.406: RN12.5 181.54,74.87 179.71,73.04 179.19,73.04 R1.C
N$474
  Top 0.406: RN11.6 RN12.3
N$475
  Top 0.406: RN12.6 182.01,74.07 179.71,71.77 176.41,71.77 R2.C
N$476
  Top 0.406: RN12.7 182.48,73.27 180.34,71.13 173.24,71.13 R3.C
N$477
  Top 0.406: RN9.4 RN10.5
N$478
  Top 0.406: RN10.6 RN9.3
N$479
  Top 0.406: RN9.2 RN10.7
N$480
  Top 0.406: RN10.8 RN9.1
N$481
  Top 0.406: RN12.2 RN11.7
N$482
  Top 0.406: RN10.1 182.81,71.06 181.61,69.86 166.89,69.86 R5.C
N$483
  Top 0.406: RN12.8 182.95,72.47 180.97,70.5 170.06,70.5 R4.C
N$484
  Top 0.406: RN10.3 183.75,69.46 182.88,68.59 160.54,68.59 R7.C
N$485
  Top 0.406: RN10.4 184.22,68.66 183.51,67.96 157.37,67.96 R8.C
N$486
  Top 0.406: RN10.2 183.28,70.26 182.25,69.23 163.72,69.23 R6.C
N$487
  Top 0.406: RN14.3 53.58,73.27 51.44,71.13 43.7,71.13 R19.C
N$488
  Top 0.406: RN14.2 53.1,74.07 50.8,71.77 46.88,71.77 R18.C
N$489
  Top 0.406: RN14.1 52.63,74.87 50.8,73.04 49.65,73.04 R17.C
N$490
  Top 0.406: RN16.4 55.31,68.66 54.61,67.96 27.82,67.96 R24.C
N$491
  Top 0.406: RN15.3 RN16.6
N$492
  Top 0.406: RN15.2 RN16.7
N$493
  Top 0.406: RN15.1 62.8,71.06 62.87,71.13 58.02,71.13 RN16.8
N$494
  Top 0.406: RN14.4 54.05,72.47 52.07,70.5 40.52,70.5 R20.C
N$495
  Top 0.406: RN16.3 54.84,69.46 53.98,68.59 31,68.59 R23.C
N$496
  Top 0.406: RN16.2 54.38,70.26 53.34,69.23 34.17,69.23 R22.C
N$497
  Top 0.406: RN16.1 53.91,71.06 52.7,69.86 37.35,69.86 R21.C
N$498  (via drill 0.6)
  Top 0.305: IC2.17 v102.87,73.67 | v219.07,73.67 219.07,74.94 219.71,75.58 v222.25,75.58 222.88,75.58 223.52,74.94 IC1.17 | U$13.B1 261.62,86.37 261.62,81.29 261.69,81.36 RN17.5 263.14,81.36 263.84,80.66 v263.84,75.58
  Bottom 0.305: v102.87,73.67 104.78,75.58 111.12,75.58 111.76,76.21 191.83,76.21 192.41,75.58 218.44,75.58 219.07,74.94 v219.07,73.67 | v222.25,75.58 v263.84,75.58
N$500
  Top 0.406: RN11.8 RN12.1
N$501
  Top 0.406: RN13.4 RN14.5
N$502
  Top 0.406: RN14.6 RN13.3
N$503
  Top 0.406: RN13.2 RN14.7
N$504
  Top 0.406: RN14.8 RN13.1
N$505
  Top 0.406: RN4.6 RN3.3
N$506
  Top 0.406: RN4.7 RN3.2
N$507
  Top 0.406: RN4.8 RN3.1
N$514
  Top 0.406: RN15.4 RN16.5
N$525  (via drill 0.5)
  Top 0.229: IC3.7 206.38,67.01 207.01,66.37 235.27,66.37 236.22,67.32 v236.22,69.99 IC1.27 | v241.3,64.47 245.03,64.47 RN18.7
  Bottom 0.229: v241.3,64.47 236.54,64.47 236.22,64.78 v236.22,69.99
N$526
  Top 0.229: IC1.28 237.49,66.37 | 237.49,66.37 236.85,65.73 205.74,65.73 205.1,66.37 IC3.8 | 237.49,66.37 237.49,64.15 238.12,63.51 245.51,63.51 RN18.8
OC_R1_A  (via drill 0.6)
  Top 0.406: IC3.18 v214,62.31 214,58.43 214.63,57.8 271.14,57.8 273.05,55.89 300.36,55.89 300.99,55.26 K1.2 | RN11.4 201.86,74.87 v202.06,74.69
  Bottom 0.406: v202.06,74.69 213.36,74.69 214,74.05 v214,62.31
OC_R1_B
  Top 0.203: RN7.5 200.73,77.55 207.33,84.15 211.77,84.15 212.72,85.1 IC4.11
  Top 0.406: IC4.11 212.72,92.72 213.36,93.36 224.16,93.36 224.79,93.99 272.42,93.99 274.7,96.28 300.1,96.28 300.99,97.17 K9.2
OC_R1_C  (via drill 0.6)
  Top 0.406: v81.28,74.94 81.21,74.87 RN13.8 | IC5.18 v93.98,62.24 93.98,60.34 95.25,59.07 144.15,59.07 144.78,58.43 K17.2
  Bottom 0.406: v81.28,74.94 92.71,74.94 93.98,73.67 v93.98,62.24
OC_R1_D
  Top 0.203: RN3.5 80.08,77.55 85.6,83.07 90.04,83.07 92.71,85.74 IC6.11
  Top 0.406: IC6.11 92.71,93.36 93.34,93.99 144.15,93.99 144.78,94.63 K25.2
OC_R2_A  (via drill 0.6)
  Top 0.406: RN11.3 200.26,74.07 v200.66,73.67 | IC3.17 v212.72,62.31 212.77,57.83 213.45,57.16 270.51,57.16 272.42,55.26 285.12,55.26 285.75,54.62 K2.2
  Bottom 0.406: v200.66,73.67 211.46,73.67 212.72,72.4 v212.72,62.31
OC_R2_B
  Top 0.203: IC4.12 211.46,85.74 210.5,84.78 207.33,84.78 200.9,78.35 RN7.6
  Top 0.406: IC4.12 211.46,93.36 212.09,93.99 223.52,93.99 224.16,94.63 271.78,94.63 274.32,97.17 285.12,97.17 285.75,97.8 K10.2
OC_R2_C  (via drill 0.6)
  Top 0.406: RN13.7 79.61,74.07 v80.01,73.67 | IC5.17 v92.71,62.24 92.71,59.07 93.98,57.8 128.91,57.8 129.54,57.16 K18.2
  Bottom 0.406: v80.01,73.67 90.17,73.67 92.71,71.13 v92.71,62.24
OC_R2_D
  Top 0.203: RN3.6 79.61,78.35 84.71,83.45 88.52,83.45 91.44,86.37 IC6.12
  Top 0.406: IC6.12 91.44,94.31 92.08,94.95 128.59,94.95 129.54,95.9 K26.2
OC_R3_A  (via drill 0.6)
  Top 0.406: RN11.2 198.52,73.27 v199.39,72.4 | IC3.16 v211.46,62.31 211.46,57.16 212.09,56.53 269.88,56.53 270.51,55.89 K3.2
  Bottom 0.406: v199.39,72.4 210.19,72.4 211.46,71.13 v211.46,62.31
OC_R3_B
  Top 0.203: RN7.7 201.06,79.15 207.33,85.42 209.87,85.42 210.19,85.74 IC4.13
  Top 0.406: IC4.13 210.19,93.99 210.82,94.63 222.88,94.63 223.52,95.26 269.88,95.26 270.51,95.9 K11.2
OC_R3_C  (via drill 0.6)
  Top 0.406: RN13.6 77.87,73.27 v78.74,72.4 | IC5.16 v91.44,62.24 91.44,57.8 92.71,56.53 113.67,56.53 114.3,55.89 K19.2
  Bottom 0.406: v78.74,72.4 88.9,72.4 91.44,69.86 v91.44,62.24
OC_R3_D
  Top 0.203: 79.14,79.15 83.82,83.83 87,83.83 90.17,87.01 IC6.13
  Top 0.229: 79.14,79.15 RN3.7
  Top 0.406: IC6.13 90.17,94.63 91.44,95.9 113.03,95.9 114.3,97.17 K27.2
OC_R4_A  (via drill 0.6)
  Top 0.406: RN11.1 196.78,72.47 v198.12,71.13 | IC3.15 v210.19,62.31 210.19,56.53 210.82,55.89 254.63,55.89 255.27,55.26 K4.2
  Bottom 0.406: v198.12,71.13 208.91,71.13 210.19,69.86 v210.19,62.31
OC_R4_B
  Top 0.203: RN7.8 201.22,79.95 207.33,86.06 208.6,86.06 208.91,86.37 IC4.14
  Top 0.406: IC4.14 208.91,94.63 209.55,95.26 222.25,95.26 222.95,95.96 254.32,95.96 255.27,96.91 K12.2
OC_R4_C  (via drill 0.6)
  Top 0.406: RN13.5 76.13,72.47 v77.47,71.13 | IC5.15 v90.17,62.24 90.17,57.16 92.08,55.26 98.42,55.26 99.06,54.62 K20.2
  Bottom 0.406: v77.47,71.13 87.63,71.13 90.17,68.59 v90.17,62.24
OC_R4_D
  Top 0.203: IC6.14 88.9,86.63 86.49,84.21 83.44,84.21 79.25,80.02 64.37,80.02
  Top 0.229: RN3.8 64.37,80.02
  Top 0.406: IC6.14 88.9,95.26 90.81,97.17 98.42,97.17 99.06,97.8 K28.2
OC_R5_A  (via drill 0.6)
  Top 0.406: RN9.8 195.65,71.06 196.85,69.86 v201.93,69.86 | IC3.14 v208.91,62.31 208.91,55.89 209.55,55.26 222.25,55.26 222.88,54.62 K5.2
  Bottom 0.406: v201.93,69.86 207.65,69.86 208.91,68.59 v208.91,62.31
OC_R5_B
  Top 0.203: IC4.15 207.65,87.01 207.33,86.69 207.01,86.69 201.68,81.36 RN6.5
  Top 0.406: IC4.15 207.65,95.26 208.28,95.9 221.62,95.9 222.88,97.17 K13.2
OC_R5_C  (via drill 0.6)
  Top 0.406: IC5.14 v88.9,62.24 88.9,57.16 87.63,55.89 67.31,55.89 66.67,55.26 K21.2 | v81.28,69.86 76.83,69.86 75.64,71.06 RN15.8
  Bottom 0.406: v81.28,69.86 87,69.86 88.9,67.96 v88.9,62.24
OC_R5_D
  Top 0.203: IC6.15 87.63,86.5 85.72,84.59 82.8,84.59 79.63,81.42 64.36,81.42
  Top 0.229: RN1.1 64.36,81.42
  Top 0.406: IC6.15 87.63,92.72 85.09,95.26 67.94,95.26 66.67,96.53 K29.2
OC_R6_A  (via drill 0.6)
  Top 0.406: RN9.7 195.18,70.26 196.85,68.59 v200.66,68.59 | IC3.13 v207.65,62.31 K6.2
  Bottom 0.406: v200.66,68.59 206.38,68.59 207.65,67.32 v207.65,62.31
OC_R6_B
  Top 0.203: RN6.6 201.53,82.16 206.38,87.01 IC4.16
  Top 0.406: IC4.16 206.38,95.9 207.65,97.17 K14.2
OC_R6_C  (via drill 0.6)
  Top 0.406: IC5.13 v87.63,62.24 87.63,58.43 86.36,57.16 52.07,57.16 51.44,56.53 K22.2 | v80.01,68.59 76.83,68.59 75.17,70.26 RN15.7
  Bottom 0.406: v80.01,68.59 86.36,68.59 87.63,67.32 v87.63,62.24
OC_R6_D
  Top 0.203: IC6.16 86.36,86.5 84.84,84.98 82.3,84.98 79.63,82.31 64.45,82.31
  Top 0.229: RN1.2 64.45,82.31
  Top 0.406: IC6.16 86.36,92.09 84.45,93.99 52.7,93.99 51.44,95.26 K30.2
OC_R7_A  (via drill 0.6)
  Top 0.406: RN9.6 194.71,69.46 196.85,67.32 v199.39,67.32 | IC3.12 v206.38,62.31 206.38,59.7 205.1,58.43 193.04,58.43 192.41,57.8 K7.2
  Bottom 0.406: v199.39,67.32 205.1,67.32 206.38,66.05 v206.38,62.31
OC_R7_B
  Top 0.203: 201.38,82.96 205.1,86.69 IC4.17
  Top 0.229: 201.38,82.96 RN6.7
  Top 0.406: IC4.17 205.1,93.36 204.47,93.99 193.04,93.99 192.41,94.63 K15.2
OC_R7_C  (via drill 0.6)
  Top 0.406: v86.36,62.24 IC5.12 86.36,61.1 86.36,59.83 84.95,58.43 36.83,58.43 36.2,57.8 K23.2 | RN15.6 74.69,69.46 76.83,67.32 v78.74,67.32
  Bottom 0.406: v78.74,67.32 85.09,67.32 86.36,66.05 v86.36,62.24
OC_R7_D
  Top 0.203: IC6.17 85.09,86.37 84.07,85.36 82.04,85.36 79.63,82.94 64.32,82.94 RN1.3
  Top 0.406: IC6.17 85.09,91.45 83.82,92.72 38.1,92.72 36.2,94.63 K31.2
OC_R8_A  (via drill 0.6)
  Top 0.406: RN9.5 194.24,68.66 196.85,66.05 v198.12,66.05 | IC3.11 v205.1,62.31 205.1,60.97 203.84,59.7 178.44,59.7 177.16,58.43 K8.2
  Bottom 0.406: v198.12,66.05 203.84,66.05 205.1,64.78 v205.1,62.31
OC_R8_B
  Top 0.203: 201.22,83.76 203.84,86.37 IC4.18
  Top 0.229: 201.22,83.76 RN6.8
  Top 0.406: IC4.18 203.84,92.09 203.2,92.72 177.8,92.72 177.16,93.36 K16.2
OC_R8_C  (via drill 0.6)
  Top 0.406: v85.09,62.24 IC5.11 85.09,65.42 84.45,66.05 82.55,66.05 81.92,65.42 81.92,60.34 81.28,59.7 21.59,59.7 20.95,59.07 K24.2 | RN15.5 74.22,68.66 76.83,66.05 v77.47,66.05
  Bottom 0.406: v77.47,66.05 83.82,66.05 85.09,64.78 v85.09,62.24
OC_R8_D
  Top 0.203: RN1.4 79.56,83.76 81.53,85.74 83.06,85.74 83.82,86.5 IC6.18
  Top 0.406: IC6.18 83.82,90.18 82.55,91.45 22.86,91.45 20.95,93.36 K32.2
REG_5V  (via drill 0.5, 0.6, 0.9)
  Top 0.254: 260.35,90.82 260.35,90.5 U$13.A2 | 313.74,30.37 312.55,30.37 v311.79,31.13 | RN26.6 RN26.5 291.72,84.7 291.72,85.23 291.34,85.61 v291.34,85.99
  Top 0.305: IC2.15 v100.33,77.48 100.97,77.48 104.14,74.31 104.14,71.13 | 224.79,77.48 226.06,78.75 226.69,78.75 227.33,79.39 | IC2.9 106.68,80.02 v105.41,78.75 | IC1.18 v224.79,76.85 | IC1.9 227.33,79.39 | 227.33,79.39 227.97,78.75 238.44,78.75 238.76,78.75 240.03,80.02 245.11,80.02 | 245.11,80.02 252.09,80.02 255.91,80.02 259.08,83.2 260.35,83.2 260.58,82.96 | 260.82,87.17 U$13.B2 U$13.A2 | C1.1 245.2,79.93 245.11,80.02 | 313.74,30.37 RNB1.6
  Top 0.406: C2.1 C3.1 124.46,71.22 124.46,69.54 | C4.1 C1.1 | IC2.18 104.14,74.31 104.78,74.94 119.15,74.94 | C8.1 119.15,74.94 | 119.15,74.94 C5.1 | C6.1 C7.1 239.8,77.71 238.76,78.75
  Top 0.61: v291.34,85.99 293.12,85.99 296.55,82.56 296.8,82.56 X26.2
  Top 0.813: 124.46,69.54 124.78,69.23 129.54,69.23 131.44,71.13 C18.+ | C3.1 124.23,69.63 123.83,69.23 119.63,69.23 119.13,69.74 119.13,71.43 C5.1 | C2.1 124.23,83.6 C19.+ | H1.1 286.23,60.18 v285.75,59.7 | IC7.4 276.99,62.37 | 276.99,62.37 v276.86,62.24 | 276.99,62.37 273.92,62.37 C10.1
  Top 1.016: C17.+ 252.09,80.02
  Top 1.27: 260.35,90.5 U$13.B2 260.35,83.51 258.76,83.51 255.59,80.34 240.03,80.34 238.44,78.75 227.65,78.75 227.33,79.07 226.38,79.07 224.79,77.48 v224.79,76.85 | H1.1 294.74,58.91 v295.27,59.32
  Bottom 0.254: 318.77,51.45 317.5,50.18 313.06,50.18 311.79,48.91 v311.79,31.13 311.79,42.56 313.06,43.83 317.5,43.83 318.77,45.1 318.77,66.69 319.4,67.32 319.4,81.93 318.77,82.56 v314.07,82.56
  Bottom 0.305: v224.79,76.85 193.68,76.85 193.04,77.48 110.49,77.48 109.86,76.85 108.58,76.85 107.95,77.48 v100.33,77.48 100.33,78.12 100.97,78.75 v105.41,78.75
  Bottom 0.61: FOR_NANO.5V 289.56,87.77 | 289.56,87.77 v291.34,85.99 | 289.56,87.77 289.56,87.64 288.93,87.01 277.5,87.01 276.23,85.74
  Bottom 0.813: v285.75,59.7 276.86,59.7 v276.86,62.24 275.59,63.51 275.59,74.31 276.86,75.58 276.86,85.1 276.23,85.74 v274.95,85.74
  Bottom 1.016: v314.07,82.56 X26.2 | v274.95,85.74 262.25,85.74 U$13.B2
REG_12V  (via drill 0.5)
  Top 0.813: BRA2.+ 301.62,63.51 299.72,60.97 292.1,60.97 288.29,64.78 286,64.78 v281.81,64.91 IC7.7 | C9.1 273.81,74.82 274.95,73.67 276.23,73.67 276.86,73.04 v276.86,67.96
  Top 1.27: C20.+ 252.09,66.69 253.37,67.96 261.62,67.96 270.51,76.85 273.61,76.85 C9.1
  Bottom 0.813: v276.86,67.96 276.86,66.05 278,64.91 v281.81,64.91
UNREG_12V  (via drill 0.6)
  Top 0.305: 179.07,76.21 R1.A
  Top 0.406: IC5.10 v83.82,62.24 | IC4.10 v214,86.06 | R8.A 152.4,76.21 | R15.A 156.21,76.21 | R6.A 160.02,76.21 | 163.83,76.21 R13.A | R4.A 167.64,76.21 | R3.A 171.45,76.21 | R2.A 175.26,76.21 | R16.A 152.4,76.21 | 152.4,76.21 156.21,76.21 | R7.A 156.21,76.21 | 156.21,76.21 160.02,76.21 | R14.A 160.02,76.21 | 160.02,76.21 163.83,76.21 | R5.A 163.83,76.21 | 163.83,76.21 167.64,76.21 | R12.A 167.64,76.21 | 167.64,76.21 171.45,76.21 | R11.A 171.45,76.21 | 171.45,76.21 175.26,76.21 | R10.A 175.26,76.21 | v93.98,90.18 IC6.10 | R24.A 22.86,76.21 | R31.A 26.67,76.21 | R30.A 30.48,76.21 | R29.A 34.29,76.21 | R28.A 38.1,76.21 | v41.91,76.21 R19.A | 45.72,76.21 R18.A | R25.A 49.53,76.21 | 49.53,76.21 R17.A | R32.A 22.86,76.21 | 22.86,76.21 26.67,76.21 | R23.A 26.67,76.21 | 26.67,76.21 30.48,76.21 | R22.A 30.48,76.21 | 30.48,76.21 34.29,76.21 | R21.A 34.29,76.21 | 34.29,76.21 38.1,76.21 | R20.A 38.1,76.21 | 38.1,76.21 v41.91,76.21 | v41.91,76.21 45.72,76.21 | R26.A 45.72,76.21 | 45.72,76.21 49.53,76.21 | R9.A 179.07,76.21 | 179.07,74.31 179.07,76.21 | 179.07,76.21 176.85,76.21 | 175.26,76.21 176.85,76.21 | 176.85,76.21 v176.85,73.04 | IC3.10 203.84,62.88 v203.8,62.31 | R27.A v41.91,76.21
  Top 2.54: BRA2.~@2 BRA2.~@1 306.02,58.43 307.28,60.2 | 307.28,60.2 U$2.TIP | X25.2 316.54,52.72 311.15,52.72 308.61,55.26 308.61,58.86 307.28,60.2
  Bottom 0.406: v214,86.06 214,94.63 213.36,95.26 | v176.85,73.04 176.85,57.16 | 203.9,57.48 204.22,57.16 | v41.91,76.21 41.91,57.16
  Bottom 0.813: v83.82,62.24 83.82,57.16 | C22.+ 15.24,87.64 | C21.+ 15.24,64.15
  Bottom 1.016: 203.9,57.48 203.8,57.48 v203.8,62.31 | C23.+ 170.81,57.16 | C24.+ 170.81,95.26
  Bottom 1.27: v93.98,90.18 93.98,95.26
  Bottom 2.54: 278.13,57.16 293.37,57.16 293.5,57.04 | 278.13,57.16 262.89,57.16 | 262.89,57.16 247.65,57.16 | 247.65,57.16 214.63,57.16 | 214.63,57.16 204.22,57.16 200.03,57.16 | 200.03,57.16 184.78,57.16 | 184.78,57.16 176.85,57.16 170.81,57.16 169.54,57.16 | 169.54,57.16 137.16,57.16 | 137.16,57.16 121.92,57.16 | 121.92,57.16 106.68,57.16 | 106.68,57.16 91.44,57.16 | 91.44,57.16 83.82,57.16 59.05,57.16 | 59.05,57.16 43.81,57.16 | 43.81,57.16 41.91,57.16 28.57,57.16 | 28.57,57.16 15.24,57.16 | 28.57,95.26 15.24,95.26 15.24,87.64 15.24,64.15 15.24,57.16 | 28.57,95.26 43.81,95.26 | 43.81,95.26 59.05,95.26 | 59.05,95.26 74.3,95.26 | 74.3,95.26 93.98,95.26 106.68,95.26 | 106.68,95.26 121.92,95.26 | 121.92,95.26 137.16,95.26 | 137.16,95.26 152.4,95.26 | 152.4,95.26 170.81,95.26 184.78,95.26 | 184.78,95.26 200.03,95.26 | 200.03,95.26 213.36,95.26 215.26,95.26 | 215.26,95.26 230.5,95.26 | 230.5,95.26 262.89,95.26 | 262.89,95.26 278.13,95.26 | K32.1 28.45,95.39 28.57,95.26 | K31.1 43.69,95.39 43.81,95.26 | K30.1 58.93,95.39 59.05,95.26 | K29.1 74.17,95.39 74.3,95.26 | K28.1 106.55,95.39 106.68,95.26 | K27.1 121.79,95.39 121.92,95.26 | K26.1 137.03,95.39 137.16,95.26 | K25.1 152.27,95.39 152.4,95.26 | K24.1 13.46,55.38 15.24,57.16 | K23.1 28.7,57.04 28.57,57.16 | K22.1 43.94,57.04 43.81,57.16 | K21.1 59.18,57.04 59.05,57.16 | K20.1 91.57,57.04 91.44,57.16 | K19.1 106.81,57.04 106.68,57.16 | K18.1 122.05,57.04 121.92,57.16 | K17.1 137.29,57.04 137.16,57.16 | K8.1 169.67,57.04 169.54,57.16 | K7.1 184.91,57.04 184.78,57.16 | K6.1 200.15,57.04 200.03,57.16 | K5.1 215.39,56.4 214.63,57.16 | K4.1 247.78,57.04 247.65,57.16 | K3.1 263.02,57.04 262.89,57.16
  Bottom 2.54: K2.1 278.26,57.04 278.13,57.16 | K1.1 293.5,57.04 | K16.1 184.66,95.39 184.78,95.26 | K15.1 199.9,95.39 200.03,95.26 | K14.1 215.14,95.39 215.26,95.26 | K13.1 230.38,95.39 230.5,95.26 | K12.1 262.76,95.39 262.89,95.26 | K11.1 278,95.39 278.13,95.26 | K9.1 308.48,99.58 305.44,96.53 293.37,96.53 | 293.37,96.53 293.37,99.58 K10.1 293.24,96.66 293.37,96.53 | 293.37,96.53 279.4,96.53 278.13,95.26 | 293.5,57.04 303.99,57.04 U$2.TIP

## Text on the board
tNames: 1 | 8 | 5 | 4 | 1 | 8 | 5 | 4 | Bank 2 | Bank 4 | ANSR32xDPDT | MCP23017 | REV.E | Address: | A1 | A2 | GND | 2016 ControlEverything.com | +5V | SC | SDA | SCL | Address A0=0 | Address A0=1 | 12V DC / Power / Supply | 12V DC / Power / Supply | 12V DC / Power / Supply | Bank 3 | Bank 1 | 8 | 5 | 4 | 1 | 8 | 5 | 4 | 1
